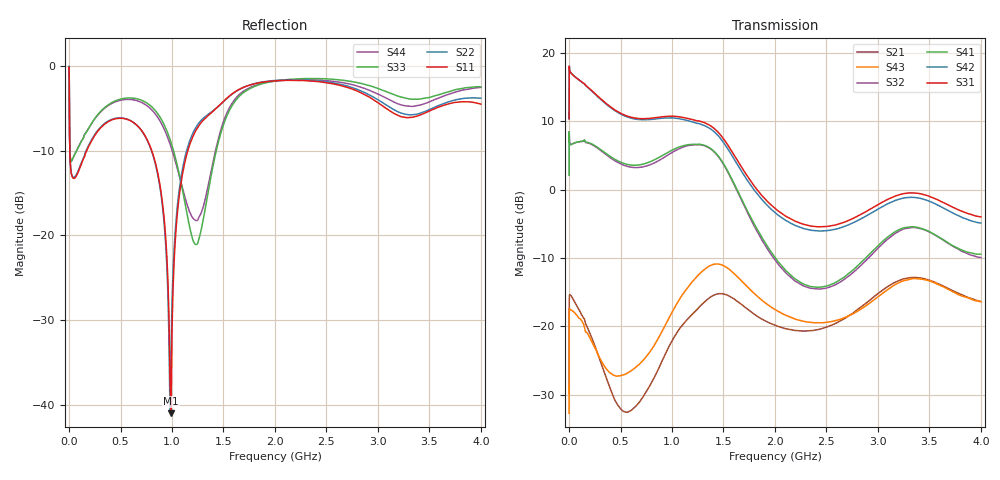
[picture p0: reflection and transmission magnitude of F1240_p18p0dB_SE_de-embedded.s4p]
! Integrated Device Technology
! Corporate Headquarters
! 6024 Silver Creek Valley Road
! San Jose, CA 95138  USA
! Phone:  1-408-284-8200
! Toll Free:  1-800-223-1366
! Webpage:  http://www.idt.com/
! Timing and RF Division
! 515 Groton Road, Suite 102
! Westford, MA 01886-6024
! Device:  F1240
! Description: Dual Intermediate Frequency Digital Variable Gain Amplifier
! Frequency:  10.0 -  500.00 MHz
! Package:  5x5 mm QFN Plastic Package: 32 pin
! Ports:  8 RF, 20 DC
!  Pin  1  = GA3 / Data  Pin 17  = RF OUT_B+
!  Pin  2  = GA4 / CLK  Pin 18  = RF OUT_B-
!  Pin  3  = GA5  Pin 19  = STBY_B
!  Pin  4  = VMODE  Pin 20  = Ground
!  Pin  5  = No Connect  Pin 21  = Ground
!  Pin  6  = GB5  Pin 22  = STB_A
!  Pin  7  = GB4  Pin 23  = RF OUT_A-  = Port 4
!  Pin  8  = GB3  Pin 24  = RF OUT_A+  = Port 3
!  Pin  9  = GB2  Pin 25  = GA0
!  Pin 10  = GB1  Pin 26  = ISET_A
!  Pin 11  = RF IN_B+  Pin 27  = VCC
!  Pin 12  = RF IN_B-  Pin 28  = Ground
!  Pin 13  = Ground  Pin 29  = RF IN_A-  = Port 2
!  Pin 14  = VCC  Pin 30  = RF IN_A+  = Port 1
!  Pin 15  = ISET_B  Pin 31  = GA1
!  Pin 16  = GB0  Pin 32  = GA2 / CSb
! Gain  = +19.5 dB
! State  = 1
! Voltage  = +5.00 V
! Current  = 85.292 mA (one channel only)
! Temperture  =  +25 C
! Test Date  =  2017-10-18
! Board  =  EB4031
! Data:  The device was measured on a custom evaluation board which has
!  individual transmission lines to the RF pins.  Data was collected
!  using a calibrated network analyzer.  The evaluation board was
!  de-embedded using Automatic Fixture Removal.
!  The reference plane is the edge of the package pin.
!  Only Channel A was measured.
!  This data is in single-ended operation.  If your needs are balanced
!  or differential S-parameters then this file needs to be used a
!  linear simulator.
! File Date:  2017-11-10  MJV
! Note:
!  Integrated Device Technology supplies this data as a sample of measured
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# Hz S dB R 100
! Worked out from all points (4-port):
!   410 points, 500 kHz to 4 GHz, reference 100 ohm
!   strongest paths, dB at 500 kHz, 930 MHz, 1.96 GHz, 2.98 GHz, 4 GHz:
!     S31: 10.4, 10.7, -2.2, -2.3, -4.0
!     S42: 10.4, 10.5, -2.8, -3.0, -4.9
!     S41: 2.1, 5.2, -9.1, -8.5, -9.4
!     S32: 2.1, 4.8, -9.4, -8.9, -9.9
!     S43: -32.7, -20.0, -17.2, -15.9, -16.4
!     S21: -29.9, -24.2, -19.6, -15.5, -16.4
!   lowest |S11| = -41.0 dB at 990 MHz (marker M1), VSWR 1.02, Z = 102 - j0.925 ohm
!   |S11| at or under -10 dB: 7.905 MHz to 171.1 MHz (163.2 MHz wide, 182 % of centre); 803 MHz to 1.153 GHz (350.4 MHz wide, 35.8 % of centre)
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500000  -0.31 -6.6  -29.75 19.5  -27.55 71.4  -62.96 68.6
        -29.90 18.9  -0.31 -6.5  -62.94 64.2  -27.57 72.5
        10.39 -105.5  2.14 72.5  -0.43 0.7  -32.78 -170.9
        2.14 73.6  10.37 -104.4  -32.75 -170.7  -0.44 3.1
3500000  -6.20 -47.9  -15.51 15.3  -21.18 7.5  -39.72 43.0
         -15.52 15.1  -6.18 -48.0  -39.68 43.0  -21.19 7.6
         17.80 -171.0  7.14 0.2  -5.84 -42.5  -17.39 27.0
         7.13 0.3  17.79 -170.8  -17.37 26.9  -5.90 -42.4
2.1e8  -9.04 -110.1  -21.25 -113.5  -24.04 -52.8  -33.28 9.2
       -21.30 -112.1  -8.91 -111.8  -33.29 9.3  -24.06 -52.8
       14.66 105.8  6.70 -61.4  -6.95 -79.7  -21.35 -124.3
       6.78 -61.3  14.60 105.0  -21.93 -123.3  -6.97 -79.1
5.6e8  -6.29 -172.6  -31.80 82.6  -25.66 -107.7  -27.47 -61.2
       -32.57 79.4  -6.27 -173.9  -27.65 -60.0  -25.84 -108.1
       10.81 20.0  3.44 -144.0  -3.79 -151.6  -26.45 82.2
       3.73 -145.0  10.68 18.8  -26.91 61.2  -3.95 -151.2
9.9e8  -41.03 -30.9  -20.62 -35.9  -22.54 163.8  -22.57 -162.7
       -22.41 -37.4  -33.74 -42.3  -22.94 -158.4  -23.00 163.3
       10.77 -83.4  5.36 124.0  -9.03 145.9  -17.35 -15.9
       5.72 119.0  10.52 -85.3  -18.23 -37.1  -9.56 151.3
1.51e9  -4.06 -139.7  -15.30 162.5  -29.67 43.1  -24.21 66.9
        -15.30 167.5  -4.09 -140.7  -24.23 72.8  -31.50 38.6
        7.25 117.5  3.46 -56.9  -6.59 -114.5  -10.94 160.2
        3.56 -61.9  6.71 115.9  -11.19 153.1  -6.23 -118.4
4e9  -4.51 -158.4  -16.39 54.8  -22.02 -34.1  -19.26 -48.1
     -16.37 54.2  -3.81 -151.6  -21.87 -29.7  -25.80 -15.1
     -3.98 -0.6  -9.93 -138.7  -2.46 -135.6  -14.69 90.2
     -9.44 -148.8  -4.88 8.4  -16.41 63.6  -2.53 -140.5
